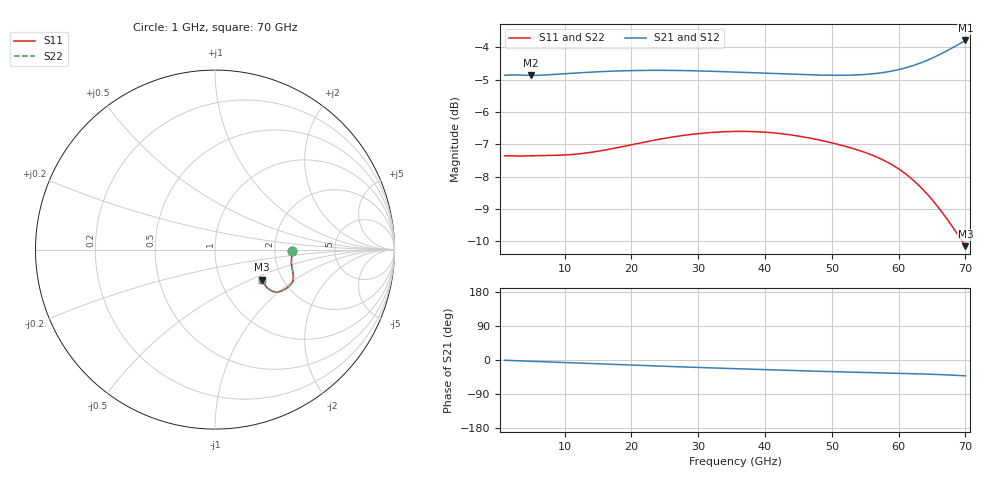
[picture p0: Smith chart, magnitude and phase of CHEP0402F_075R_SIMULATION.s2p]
! Touchstone file exported from HFSS 2026.1.0
!  File:  S:/COMPOSANTS_3D_CRYPTES/CHEP0402F/2026R1/PCB_&_COMP/PCB_V1.1.003_CHEP0402F_V1.aedt
!  $RV = 75ohm
# GHz S MA R 50.000000
! Terminal data exported
! Port[1] = LINE_T1
! Port[2] = LINE_T2
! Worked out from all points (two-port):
!   401 points, 1 GHz to 70 GHz, reference 50 ohm
!   highest |S21| = -3.78 dB at 70 GHz (marker M1); lowest = -4.9 dB at 4.968 GHz (marker M2)
!   |S21| within 3 dB of the highest: start of sweep to end of sweep
!   lowest |S11| = -10.2 dB at 70 GHz (marker M3), VSWR 1.90, Z = 78.7 - j29.3 ohm
!   |S11| at or under -10 dB: 69.52 GHz to end of sweep
!   |S22| runs from -10.2 to -6.6 dB; largest |S21 - S12| = 2.5e-14
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1  0.4287 -0.9  0.5713 -0.7  0.5713 -0.7  0.4287 -0.9
4.9675  0.4287 -4.1  0.5711 -3.4  0.5711 -3.4  0.4287 -4.0
9.4525  0.4298 -7.7  0.5739 -6.2  0.5739 -6.2  0.4297 -7.7
12.5575  0.4323 -9.9  0.5767 -8.3  0.5767 -8.3  0.4321 -9.9
18.25  0.4422 -13.6  0.5804 -12.2  0.5804 -12.2  0.442 -13.6
24.115  0.4548 -16.9  0.5815 -16.1  0.5815 -16.1  0.4545 -16.8
30.1525  0.4642 -19.7  0.5803 -19.8  0.5803 -19.8  0.4641 -19.7
35.5  0.4677 -22.0  0.5779 -22.9  0.5779 -22.9  0.4676 -22.0
41.1925  0.4654 -24.6  0.575 -26.1  0.575 -26.1  0.4654 -24.5
47.0575  0.4559 -27.7  0.5721 -29.3  0.5721 -29.3  0.456 -27.6
50.68  0.4472 -29.7  0.5713 -31.1  0.5713 -31.1  0.4473 -29.6
53.9575  0.4375 -31.7  0.5722 -32.5  0.5722 -32.5  0.4375 -31.6
56.545  0.4277 -33.2  0.5749 -33.6  0.5749 -33.6  0.4277 -33.1
58.615  0.4176 -34.4  0.579 -34.5  0.579 -34.5  0.4176 -34.3
61.5475  0.3982 -35.8  0.5887 -35.8  0.5887 -35.8  0.3982 -35.7
62.9275  0.3868 -36.2  0.5951 -36.4  0.5951 -36.4  0.3868 -36.1
64.3075  0.3738 -36.3  0.6028 -37.2  0.6028 -37.2  0.3739 -36.2
65.515  0.3614 -36.2  0.6106 -38.0  0.6106 -38.0  0.3615 -36.1
66.895  0.3463 -35.7  0.6208 -39.0  0.6208 -39.0  0.3464 -35.5
68.275  0.3306 -34.7  0.6319 -40.1  0.6319 -40.1  0.3306 -34.6
69.655  0.3146 -33.2  0.6438 -41.5  0.6438 -41.5  0.3147 -33.1
70  0.3107 -32.8  0.6468 -41.8  0.6468 -41.8  0.3108 -32.7
